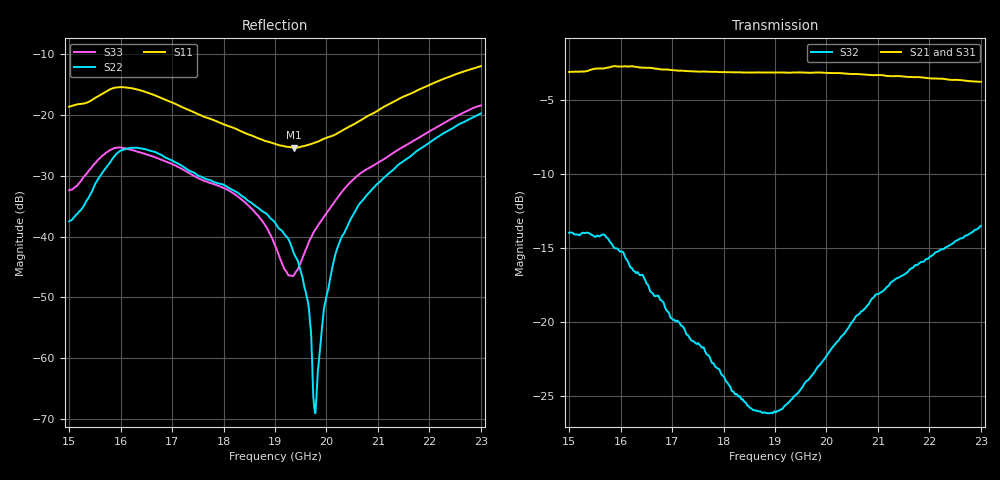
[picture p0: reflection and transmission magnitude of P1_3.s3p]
!The following data was pulled from an Agilent PNA
!This sNp file was generated from the data in the RF Test software
!NOTE:  Smoothing/Math/Corrections applied on any given trace ARE included in the data saved here
# MHz S dB R 50
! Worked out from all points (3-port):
!   1601 points, 15 GHz to 23 GHz, reference 50 ohm
!   strongest paths, dB at 15 GHz, 17 GHz, 19 GHz, 21 GHz, 23 GHz:
!     S21: -3.1, -2.9, -3.1, -3.3, -3.7
!     S31: -2.8, -3.1, -3.1, -3.4, -3.8
!     S32: -14.0, -19.8, -26.1, -18.1, -13.5
!   lowest |S11| = -25.4 dB at 19.37 GHz (marker M1), VSWR 1.11, Z = 50 - j5.41 ohm
!   |S11| at or under -10 dB: start of sweep to end of sweep
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15000  -18.61 49.8  -3.10 -168.7  -2.89 -171.1
       -3.07 -168.4  -37.47 108.1  -14.01 148.4
       -2.81 -170.8  -13.97 148.4  -32.37 137.4
15570  -16.85 51.6  -2.90 -175.5  -3.00 10.7
       -2.84 -175.7  -30.43 95.6  -14.21 134.7
       -2.92 -10.6  -14.19 134.8  -27.30 105.2
15665  -16.39 50.0  -2.84 -176.9  -3.02 178.5
       -2.83 -176.8  -29.25 91.2  -14.18 131.0
       -2.91 178.7  -14.08 131.2  -26.57 97.7
15855  -15.55 42.8  -2.82 10.3  -3.16 175.5
       -2.70 -10.4  -27.03 79.4  -14.92 123.8
       -3.00 175.4  -14.89 123.2  -25.51 82.0
15940  -15.42 38.8  -2.81 178.5  -3.21 174.6
       -2.71 178.6  -26.22 71.5  -15.06 120.7
       -3.09 174.6  -15.04 120.5  -25.33 74.4
19000  -24.72 -63.8  -3.16 136.8  -3.16 134.9
       -3.12 136.2  -37.70 -7.3  -26.06 7.1
       -3.15 133.9  -26.09 6.7  -41.42 23.0
19370  -25.35 -87.1  -3.13 131.4  -3.12 129.2
       -3.11 131.0  -42.81 -12.8  -25.02 -17.6
       -3.13 128.8  -25.05 -17.7  -46.30 88.4
19780  -24.49 -113.9  -3.13 125.3  -3.13 122.9
       -3.11 125.1  -69.01 -46.3  -23.31 -41.6
       -3.12 122.5  -23.33 -41.7  -38.87 133.5
20600  -21.15 -153.1  -3.23 112.6  -3.27 109.9
       -3.21 112.8  -35.15 162.5  -19.55 -76.8
       -3.26 110.2  -19.55 -76.8  -30.00 142.2
23000  -11.94 152.8  -3.79 77.5  -3.80 74.7
       -3.74 77.6  -19.73 132.5  -13.42 -133.0
       -3.82 74.8  -13.49 -133.0  -18.41 129.3
